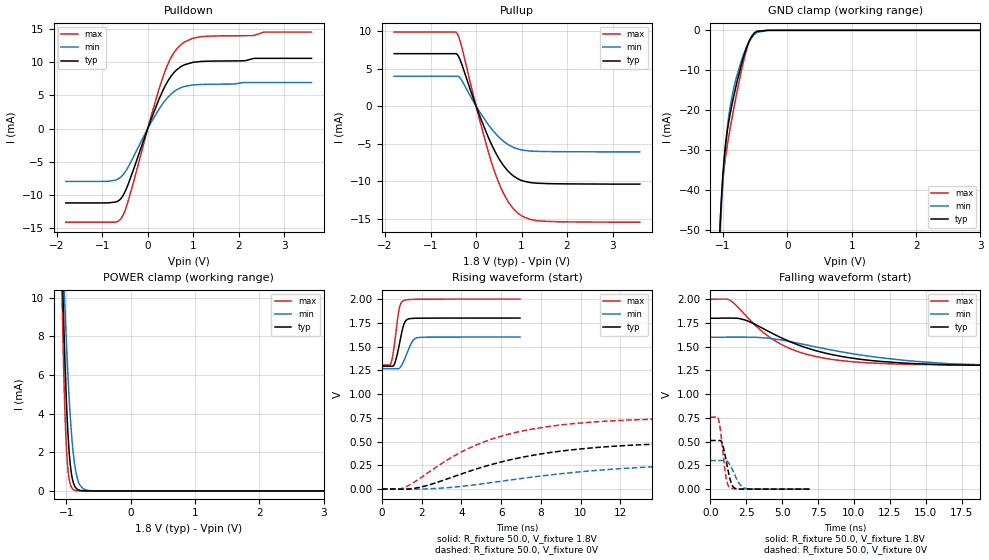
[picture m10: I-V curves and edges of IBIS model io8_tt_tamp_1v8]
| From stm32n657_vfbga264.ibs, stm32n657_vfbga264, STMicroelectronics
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[Model]   io8_tt_tamp_1v8
Model_type I/O
Polarity   Non-Inverting
Enable   Active-Low
| CAP_THRESHOLD on pad IOTT is "UDTCAPC" :
| Rising=30.0% of vddiov33m   Falling=70.0% of vddiov33m
| C_comp min and max val. don't necessarily correlate with the min and max pvt
| but are the smallest and greatest pad capacitance found.
| var   typ   min   max
C_comp   1.44560pF  1.40495pF  1.47163pF
|C_comp_pullup   766.56000fF  743.21000fF  784.07000fF
|C_comp_pulldown   679.03555fF  661.73500fF  687.55750fF
Vinl = 480.0mV
Vinh = 1.4V
Vmeas = 900.0mV   | Reference voltage for timing measurements
Cref  = 50.0pF   | Timing specification test load capacitance value
Rref  = 100.0MOhm   | Timing specification test load resistance value
Vref  = 900.0mV   | Timing specification test load voltage
[Model Spec]
| TIME_THRESHOLD on pin ZIV08SW is "CMOS" :
| Rising=50.0% of vddv08sw   Falling=50.0% of vddv08sw
Vinl 1.07470V 960.70000mV 1.21270V
Vinh 1.54130V 1.38830V 1.71030V
| variable   typ   min   max
[Temperature Range] 25.0 125.0 -40.0
| variable   typ   min   max
[Voltage Range] 1.8V 1.6V 2.0V
| variable   typ   min   max
[POWER Clamp Reference] 1.8V 1.6V 2.0V
| variable   typ   min   max
[GND Clamp Reference] 0V 0V 0V
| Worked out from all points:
|   slope of the pulldown table from 0 to 0.27 V, typ, clamps not added: 56.7 ohm
|   slope of the pullup table from 0 to 0.27 V, typ, clamps not added: 64.9 ohm
|   GND clamp passes 1 mA (typ) near -0.53 V on its own axis
|   POWER clamp passes 1 mA (typ) near -0.93 V on its own axis
|   rising waveform, R_fixture 50.0, V_fixture 1.8V: 20-80 % time 310ps typ, 407ps min, 263ps max; typ from 1.29 V to 1.8 V
|   falling waveform, R_fixture 50.0, V_fixture 1.8V: 20-80 % time 5.67ns typ, 9.23ns min, 3.92ns max; typ from 1.8 V to 1.29 V
|   rising waveform, R_fixture 50.0, V_fixture 0V: 20-80 % time 6.24ns typ, 9.14ns min, 4.79ns max; typ from 0 V to 0.513 V
|   falling waveform, R_fixture 50.0, V_fixture 0V: 20-80 % time 426ps typ, 600ps min, 351ps max; typ from 0.513 V to 0 V
[POWER Clamp]
-1.8V     154.4mA    107.1mA    224.4mA
-1.07V    12.25mA    13.82mA    10.53mA
-1.05V    9.71mA     11.92mA    7.356mA
-1.03V    7.448mA    10.14mA    4.813mA
-1.01V    5.5mA      8.481mA    2.941mA
-990mV    3.897mA    6.961mA    1.686mA
-970mV    2.647mA    5.595mA    919.8uA
-940mV    1.378mA    3.863mA    349.2uA
-880mV    312.8uA    1.571mA    46.18uA
-790mV    28.88uA    303.2uA    2.148uA
-610mV    214.2nA    7.645uA    15.6nA
3.6V      0A         0A         0A
[GND Clamp]
-1.8V     -1.248A    -1.23A     -1.258A
-1.05V    -50.38mA   -53.43mA   -50.32mA
-1.04V    -46.6mA    -49.44mA   -46.84mA
-1.01V    -37.75mA   -39.7mA    -39.15mA
-970mV    -29.9mA    -30.41mA   -32.79mA
-920mV    -23.69mA   -22.57mA   -27.38mA
-870mV    -19.26mA   -17.32mA   -22.78mA
-780mV    -12.71mA   -11.05mA   -15.14mA
-650mV    -4.993mA   -4.772mA   -5.76mA
-570mV    -1.936mA   -2.222mA   -2.04mA
-480mV    -339.6uA   -627.3uA   -256uA
3.6V      78.07nA    2.857uA    15.87nA
| variable   typ   min   max
[Pullup Reference] 1.8V 1.6V 2.0V
| variable   typ   min   max
[Pulldown Reference] 0V 0V 0V
[Pullup]
-1.8V     6.977mA    3.977mA    9.855mA
-420mV    6.911mA    3.977mA    9.716mA
-330mV    5.842mA    3.568mA    8.232mA
70mV      -1.149mA   -695.4uA   -1.66mA
250mV     -3.883mA   -2.32mA    -5.669mA
410mV     -5.971mA   -3.54mA    -8.759mA
540mV     -7.355mA   -4.351mA   -10.8mA
670mV     -8.429mA   -4.985mA   -12.37mA
960mV     -9.808mA   -5.787mA   -14.45mA
1.18V     -10.18mA   -5.983mA   -15.08mA
1.56V     -10.33mA   -6.062mA   -15.37mA
3.6V      -10.4mA    -6.102mA   -15.47mA
[Pulldown]
-1.8V     -11.16mA   -7.923mA   -14.05mA
-870mV    -11.15mA   -7.921mA   -14.05mA
-670mV    -10.94mA   -7.621mA   -13.98mA
-570mV    -10.34mA   -7.128mA   -13.35mA
-420mV    -8.184mA   -5.644mA   -10.66mA
70mV      1.323mA    886.5uA    1.768mA
330mV     5.679mA    3.752mA    7.67mA
530mV     8.038mA    5.297mA    10.89mA
760mV     9.438mA    6.239mA    12.79mA
1.18V     10.11mA    6.643mA    13.83mA
2.55V     10.57mA    6.932mA    14.51mA
3.6V      10.57mA    6.932mA    14.51mA
[Ramp]
dV/dt_r 307.60806mV/6.23427ns 180.7401mV/9.04868ns 455.17025mV/4.79145ns
dV/dt_f 304.14433mV/5.67197ns 199.72249mV/9.12703ns 416.82094mV/3.91989ns
R_load = 50.0
| Removed startup time: 0s 0s 0s  .
| Removed end time: 6.95ns.
[Rising Waveform]
R_fixture   = 50.0
V_fixture   = 1.8V
V_fixture_min = 1.6V
V_fixture_max = 2.0V
0s        1.293V     1.267V     1.305V
450ps     1.293V     1.267V     1.317V
550ps     1.292V     1.267V     1.407V
650ps     1.324V     1.267V     1.55V
850ps     1.492V     1.267V     1.874V
950ps     1.597V     1.287V     1.952V
1.1ns     1.73V      1.347V     1.985V
1.5ns     1.796V     1.542V     1.996V
1.8ns     1.798V     1.593V     1.998V
6.95ns    1.8V       1.6V       2V
| Removed startup time: 0s 0s 0s  .
| Removed end time: 74.9ns.
[Falling Waveform]
R_fixture   = 50.0
V_fixture   = 1.8V
V_fixture_min = 1.6V
V_fixture_max = 2.0V
0s        1.8V       1.6V       2V
1.4ns     1.802V     1.601V     1.987V
2.4ns     1.782V     1.601V     1.841V
3.8ns     1.682V     1.593V     1.638V
5.6ns     1.55V      1.553V     1.478V
7.7ns     1.445V     1.487V     1.386V
10.6ns    1.365V     1.41V      1.334V
16.7ns    1.309V     1.321V     1.309V
25ns      1.295V     1.281V     1.306V
74.9ns    1.293V     1.267V     1.305V
| Removed startup time: 0s 0s 0s  .
| Removed end time: 74.9ns.
[Rising Waveform]
R_fixture   = 50.0
V_fixture   = 0V
V_fixture_min = 0V
V_fixture_max = 0V
0s        349.4nV    4.736uV    499.3nV
900ps     -1.253mV   -593.2uV   -579.2uV
1.2ns     -894.9uV   -845uV     22.71mV
2.2ns     33.26mV    603.6uV    152.8mV
4ns       158.4mV    27.72mV    389.6mV
6.1ns     289.7mV    84.3mV     561.4mV
8.7ns     390.3mV    153.8mV    666.5mV
12.2ns    457.1mV    217.1mV    723.9mV
25ns      508.9mV    289.1mV    757.5mV
74.9ns    512.7mV    301.2mV    758.6mV
| Removed startup time: 0s 0s 0s  .
| Removed end time: 6.95ns.
[Falling Waveform]
R_fixture   = 50.0
V_fixture   = 0V
V_fixture_min = 0V
V_fixture_max = 0V
0s        512.7mV    301.3mV    758.6mV
500ps     512.7mV    301.3mV    759.7mV
600ps     512.6mV    301.3mV    724.1mV
800ps     494.8mV    301.3mV    509.5mV
1.1ns     308.4mV    301.7mV    125.1mV
1.35ns    123.2mV    260.5mV    19.16mV
1.65ns    16.31mV    170.4mV    5.425mV
2.05ns    1.623mV    54.52mV    2.326mV
2.45ns    684.4uV    8.059mV    1.315mV
6.95ns    85.69uV    81.79uV    136.2uV
